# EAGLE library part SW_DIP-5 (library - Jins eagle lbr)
DIP SWITCH
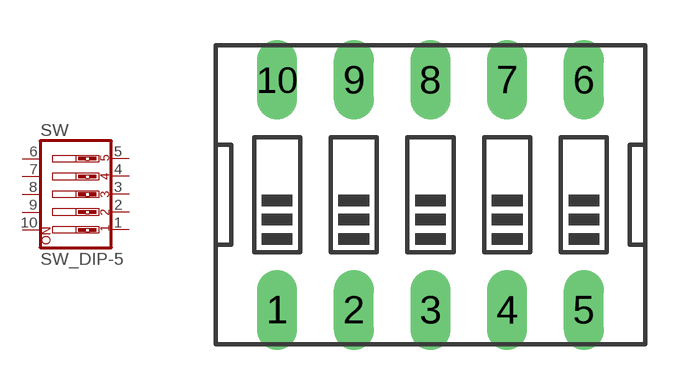
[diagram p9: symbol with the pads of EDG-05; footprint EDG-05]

Designator prefix SW

## SW_DIP-5  [EDG-05]
1  1  pas
2  2  pas
3  3  pas
4  4  pas
5  5  pas
6  6  pas
7  7  pas
8  8  pas
9  9  pas
10  10  pas

## Footprint EDG-05 (pad centres in mm)
DIP SWITCH
drill 0.813 long: 1 -5.08,-3.81; 2 -2.54,-3.81; 3 0,-3.81; 4 2.54,-3.81; 5 5.08,-3.81; 6 5.08,3.81; 7 2.54,3.81; 8 0,3.81; 9 -2.54,3.81; 10 -5.08,3.81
